PROGRAM MAIN
VAR
	DRAND1:DRAND;                     //声明随机函数功能块
	TON1:TON;                         //声明时间函数功能块
	a:INT;                            //声明随机函数的输入变量
	real_data:LREAL;                  //声明随机函数的输出变量
	array100:ARRAY[0..99]OF LREAL;    //声明Scope项目所需要采集的数组变量
	m:INT;                            //声明数组中的元素变量
END_VAR

DRAND1(Seed:=a,Num=>real_data);            //随机生成数

TON1(IN:=NOT ton1.q,PT:=T#10MS,Q=>,ET=>);  //刷新时间(10ms)

IF ton1.Q THEN
	array100[m]:=real_data;
	IF m<100 THEN
		m:=m+1;
	ELSE                                   
		m:=1;
	END_IF                 
END_IF                                     //每刷新10ms,将随机生成的数从0-99依次赋值给数组中的元素

END_PROGRAM
